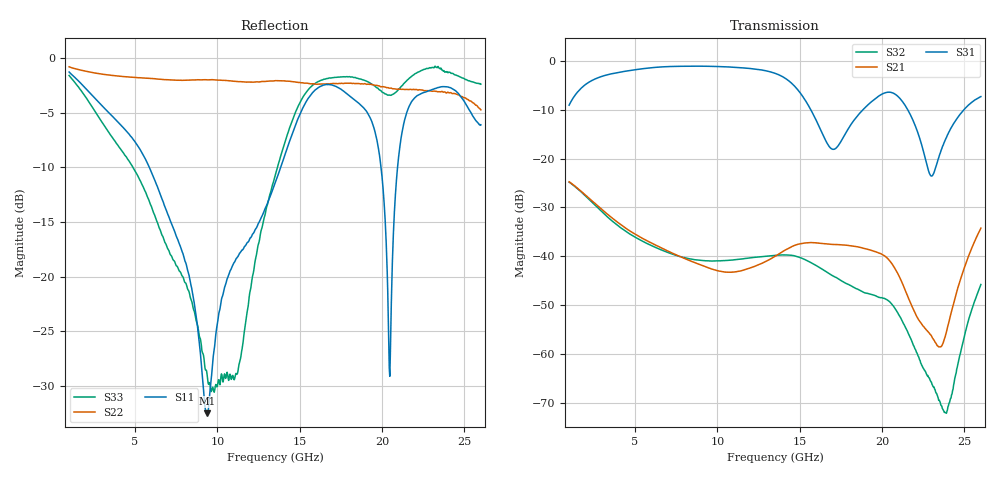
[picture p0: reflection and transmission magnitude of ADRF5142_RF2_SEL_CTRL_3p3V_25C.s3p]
! Device: ADRF5142
! Description: Silicon, SPDT Switch, Reflective
! Frequency: 8.00 GHz - 11.00 GHz
! Ports:
!  RFC = Port 1
!  RF1 = Port 2
!  RF2 = Port 3
! VDD = +3.3V
! VSS = -3.3V
! CTRL = +3.3V
! Temp = 25C
! Data:  Data was collected using an calibrated 4 port network analyzer.
!  The reference plane is the package pins of ADRF5142 switch.
! Notes: Analog Devices supplies this data as a sample of measured data
!  for this product.  Your particular data for this product may vary.
!  Data was taken at 25 degrees C.
!  Analog Devices reserves the right to change this data at anytime.
# HZ S DB R 50
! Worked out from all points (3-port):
!   801 points, 1 GHz to 26 GHz, reference 50 ohm
!   strongest paths, dB at 1 GHz, 7.25 GHz, 13.5 GHz, 19.75 GHz, 26 GHz:
!     S31: -9.1, -1.1, -2.5, -7.3, -7.3
!     S21: -24.7, -39.3, -40.0, -39.3, -34.2
!     S32: -24.8, -39.5, -39.8, -48.3, -45.8
!   lowest |S11| = -32.5 dB at 9.375 GHz (marker M1), VSWR 1.05, Z = 51.2 - j2.08 ohm
!   |S11| at or under -10 dB: 5.866 GHz to 13.84 GHz (7.977 GHz wide, 80.9 % of centre); 19.93 GHz to 20.94 GHz (1.007 GHz wide, 4.93 % of centre)
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1e9  -1.29 158.0  -24.75 -39.2  -9.05 37.6
     -24.75 -39.2  -0.82 171.0  -24.81 -56.8
     -9.05 37.6  -24.81 -56.8  -1.61 124.7
5.9062e9  -10.14 94.5  -37.11 -120.3  -1.41 -87.1
          -37.11 -120.3  -1.88 141.6  -37.65 140.9
          -1.41 -87.1  -37.65 140.9  -13.29 -73.4
9.375e9  -32.51 -59.1  -42.27 -143.9  -1.08 -165.0
         -42.27 -143.9  -2.01 119.2  -40.93 68.7
         -1.08 -165.0  -40.93 68.7  -28.93 -109.9
1.35e10  -11.48 -121.5  -40.01 -156.5  -2.53 91.1
         -40.01 -156.5  -2.09 93.8  -39.81 -27.1
         -2.53 91.1  -39.81 -27.1  -10.77 69.5
1.58125e10  -3.13 -175.9  -37.21 155.6  -10.87 26.2
            -37.21 155.6  -2.37 79.8  -41.55 -105.6
            -10.87 26.2  -41.55 -105.6  -2.47 -21.1
1.89687e10  -4.73 90.9  -38.44 91.4  -9.54 61.9
            -38.44 91.4  -2.36 59.8  -47.50 156.9
            -9.54 61.9  -47.50 156.9  -2.09 -99.1
2.04687e10  -29.13 -58.4  -40.93 50.9  -6.40 9.2
            -40.93 50.9  -2.78 50.4  -49.32 94.4
            -6.40 9.2  -49.32 94.4  -3.41 -112.9
2.19062e10  -3.79 157.6  -50.90 37.5  -12.37 -49.5
            -50.90 37.5  -2.88 37.8  -58.26 32.2
            -12.37 -49.5  -58.26 32.2  -1.57 -129.2
2.38437e10  -2.63 68.1  -56.31 154.6  -16.09 23.5
            -56.31 154.6  -3.14 25.3  -72.02 -39.3
            -16.09 23.5  -72.02 -39.3  -1.28 -160.2
2.6e10  -6.13 -24.4  -34.23 156.6  -7.29 -25.6
        -34.23 156.6  -4.76 12.7  -45.78 167.8
        -7.29 -25.6  -45.78 167.8  -2.40 160.7
